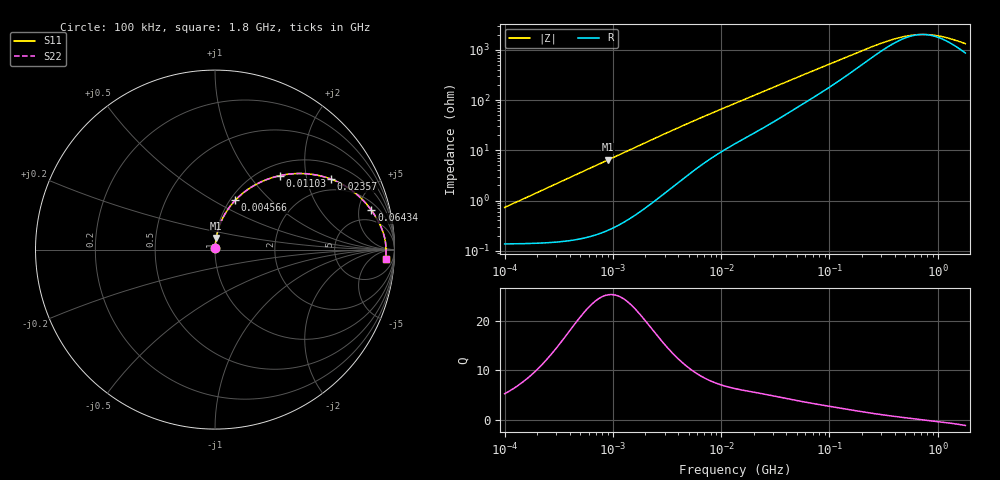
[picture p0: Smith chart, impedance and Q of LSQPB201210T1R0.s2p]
! LSQPB201210T1R0  S-PARAMETER MODEL  ( General Type )
! Model Generated by TAIYO YUDEN Corporation (http://www.ty-top.com)
! Version 2.0
! TAIYO YUDEN Control No. 100810NF18SB-HKC
! Copyright(c) 2007 TAIYO YUDEN CO.,LTD. All Rights Reserved.
! Product Description (link to TY-COMPAS)
! https://ds.yuden.co.jp/TYCOMPAS/or/detail?pn=LSQPB201210T1R0M&u=M
! Products Name : Inductors
! Characteristics :
!  Inductance : 1.0 uH , SRF(min) : 300 MHz , DC Resistance(max) : 0.1755 Ohm
!  Rated Current : Saturation :850 mA , Temp Rise : 850 mA (40 degC)
!  Case Size : 2.0 x 1.25 / 0.079 x 0.049 [mm/inch] , Thickness : 1.0 / 0.04 [mm/inch]
!  (Conditions: Temperature = 25 degC , DC Bias Current/Voltage = 0A / 0V)
! External Node Assignments :
!  1  o---GGG---o  2
! GND o---------o GND
! Frequency Range : 0.1MHz  -  1800MHz  [ 402 STEP ]
# MHz S RI R 50
! Freq[MHz].  S11 Real  S11 Imag  S21 Real  S21 Imag  S12 Real  S12 Imag  S22 Real  S22 Imag
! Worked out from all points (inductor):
!   401 points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, 100 kHz to 1.8 GHz, reference 50 ohm
!   read as one part in series: L = 1.14 uH near 105 kHz
!   highest Q = 25.3 at 906.6 kHz (marker M1), where L = 1.14 uH
!   self-resonance near 717.9 MHz
!   S11 on the Smith chart (normalised r, x): 100 kHz: 1.00, +0.01; 4.566 MHz: 1.06, +0.64; 11.03 MHz: 1.21, +1.43; 23.57 MHz: 1.53, +2.82; 64.34 MHz: 2.98, +6.78; 1.8 GHz: 18, -20
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0.1  0.00141 0.00714  0.9986 -0.00714  0.9986 -0.00714  0.00141 0.00714
0.516129  0.0031 0.0368  0.9969 -0.0368  0.9969 -0.0368  0.0031 0.0368
0.906643  0.00671 0.0643  0.9933 -0.0643  0.9933 -0.0643  0.00671 0.0643
1.592628  0.0176 0.1111  0.9824 -0.1111  0.9824 -0.1111  0.0176 0.1111
2.66389  0.0445 0.1783  0.9555 -0.1783  0.9555 -0.1783  0.0445 0.1783
4.566214  0.1123 0.2743  0.8877 -0.2743  0.8877 -0.2743  0.1123 0.2743
6.92477  0.2086 0.3517  0.7914 -0.3517  0.7914 -0.3517  0.2086 0.3517
11.02886  0.3619 0.4122  0.6381 -0.4122  0.6381 -0.4122  0.3619 0.4122
13.41641  0.436 0.4228  0.564 -0.4228  0.564 -0.4228  0.436 0.4228
17.56533  0.5401 0.4195  0.4599 -0.4195  0.4599 -0.4195  0.5401 0.4195
23.56755  0.647 0.3925  0.353 -0.3925  0.353 -0.3925  0.647 0.3925
38.46609  0.7855 0.3116  0.2145 -0.3116  0.2145 -0.3116  0.7855 0.3116
64.33982  0.8713 0.2194  0.1287 -0.2194  0.1287 -0.2194  0.8713 0.2194
69.24595  0.8797 0.2075  0.1203 -0.2075  0.1203 -0.2075  0.8797 0.2075
151.6408  0.9335 0.1047  0.0665 -0.1047  0.0665 -0.1047  0.9335 0.1047
253.6402  0.9464 0.0595  0.0536 -0.0595  0.0536 -0.0595  0.9464 0.0595
357.3983  0.9503 0.0367  0.0497 -0.0367  0.0497 -0.0367  0.9503 0.0367
542.0029  0.9525 0.0139  0.0475 -0.0139  0.0475 -0.0139  0.9525 0.0139
659.3364  0.9529 0.00417  0.0471 -0.00417  0.0471 -0.00417  0.9529 0.00417
782.6622  0.9531 -0.00425  0.0469 0.00425  0.0469 0.00425  0.9531 -0.00425
1130.179  0.9528 -0.0231  0.0472 0.0231  0.0472 0.0231  0.9528 -0.0231
1800  0.9506 -0.0517  0.0494 0.0517  0.0494 0.0517  0.9506 -0.0517
